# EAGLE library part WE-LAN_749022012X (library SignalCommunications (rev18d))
WE-LAN LAN Transformer Characteristics Compliant with standards: IEEE 802.3u, IEEE 802.3ab, IEEE 802.3af, IEEE 802.3at and upcoming IEE 802.3bt SMD Applications Ethernet speed up to 10 Gbit/s Power over Ethernet PoE and PoE+ Compliant with most IC’s for Ethernet applications such as Intel, AMD, Microchip and Realtek Hub, Router, Switches, IPcameras, IoT Details see: http://katalog.we-online.de/en/pbs/WE-LAN Created by Yingchun Shan 2016 (C) Wurth Elektronik
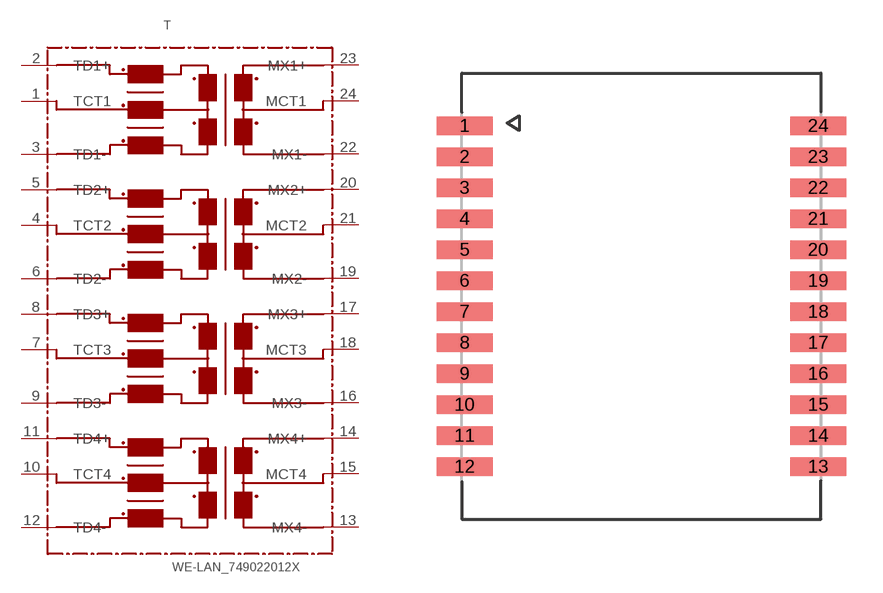
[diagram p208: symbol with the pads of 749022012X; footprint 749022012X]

Designator prefix T

## WE-LAN_749022012X_7490220120, WE-LAN_749022012X_7490220121, WE-LAN_749022012X_7490220122, WE-LAN_749022012X_7490220123  [749022012X]
1  TCT1
2  TD1+
3  TD1-
4  TCT2
5  TD2+
6  TD2-
7  TCT3
8  TD3+
9  TD3-
10  TCT4
11  TD4+
12  TD4-
13  MX4-
14  MX4+
15  MCT4
16  MX3-
17  MX3+
18  MCT3
19  MX2-
20  MX2+
21  MCT2
22  MX1-
23  MX1+
24  MCT1

## Footprint 749022012X (pad centres in mm)
smd 2.29 x 0.76: 1 -7.24,6.985; 2 -7.24,5.715; 3 -7.24,4.445; 4 -7.24,3.175; 5 -7.24,1.905; 6 -7.24,0.635; 7 -7.24,-0.635; 8 -7.24,-1.905; 9 -7.24,-3.175; 10 -7.24,-4.445; 11 -7.24,-5.715; 12 -7.24,-6.985; 13 7.24,-6.985; 14 7.24,-5.715; 15 7.24,-4.445; 16 7.24,-3.175; 17 7.24,-1.905; 18 7.24,-0.635; 19 7.24,0.635; 20 7.24,1.905; 21 7.24,3.175; 22 7.24,4.445; 23 7.24,5.715; 24 7.24,6.985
